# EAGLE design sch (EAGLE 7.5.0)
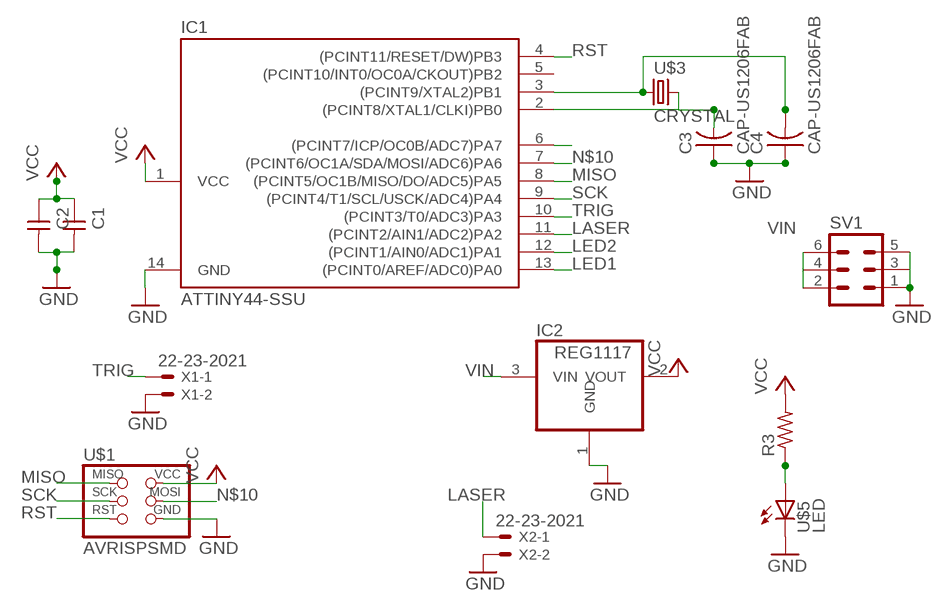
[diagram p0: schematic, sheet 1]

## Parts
C1  CAP-UNPOLARIZEDFAB  [C1206FAB]
C2  CAP-UNPOLARIZEDFAB  [C1206FAB]
C3  CAP-US1206FAB  [C1206FAB]
C4  CAP-US1206FAB  [C1206FAB]
IC1  ATTINY44-SSU  [SOIC14]
IC2  REG1117  [SOT223]
R3  RES-US1206FAB  [R1206FAB]
SV1  MA03-2  [MA03-2]
U$1  AVRISPSMD  [2X03SMD]
U$3  CRYSTAL  [2-SMD-5X3MM]
U$5  LED  [LED1206]
X1  22-23-2021  [22-23-2021]
X2  22-23-2021  [22-23-2021]

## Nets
GND: IC2.1(GND) SV1.1 SV1.3 SV1.5 X1.2 X2.2
K1: IC1.6((PCINT7/ICP/OC0B/ADC7)PA7) R3.1 U$5.1(A)
LASER: IC1.11((PCINT2/AIN1/ADC2)PA2) X2.1
LED1: IC1.13((PCINT0/AREF/ADC0)PA0)
LED2: IC1.12((PCINT1/AIN0/ADC1)PA1)
MISO: IC1.8((PCINT5/OC1B/MISO/DO/ADC5)PA5) U$1.1(MISO)
N$3: C4.2 IC1.3((PCINT9/XTAL2)PB1) U$3.P$1
N$5: C3.2 IC1.2((PCINT8/XTAL1/CLKI)PB0) U$3.P$2
N$6: C1.2 C2.2 C3.1 C4.1 IC1.14(GND) U$1.6(GND) U$5.2(C) ; supply symbol labelled GND
N$9: C1.1 C2.1 IC1.1(VCC) IC2.2(VOUT) R3.2 U$1.2(VCC) ; supply symbol labelled VCC
N$10: IC1.7((PCINT6/OC1A/SDA/MOSI/ADC6)PA6) U$1.4(MOSI)
RST: IC1.4((PCINT11/RESET/DW)PB3) U$1.5(RST)
SCK: IC1.9((PCINT4/T1/SCL/USCK/ADC4)PA4) U$1.3(SCK)
TRIG: IC1.10((PCINT3/T0/ADC3)PA3) X1.1
VIN: IC2.3(VIN) SV1.2 SV1.4 SV1.6
Unconnected: IC1.5((PCINT10/INT0/OC0A/CKOUT)PB2)

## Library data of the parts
C1 C2 = fab:CAP-UNPOLARIZED
C3 C4 = fab:CAP-US
IC1 = fab:ATTINY44
IC2 = burr-brown:REG1117: 800mA and 1A Low Dropout (LDO) Positive Regulator 1.8V, 2.5V, 2.85V, 3.3V, 5V, and Adj; MPN: REG1117; OC_FARNELL: 1097566; OC_NEWARK: 14P6981
R3 = fab:RES-US: Resistor (US Symbol)
SV1 = con-lstb:MA03-2: PIN HEADER; OC_FARNELL: unknown; OC_NEWARK: unknown
U$1 = fab:AVRISP
U$3 = fab:CRYSTAL
U$5 = fab:LED: LED
X1 X2 = con-molex:22-23-2021: .100" (2.54mm) Center Header - 2 Pin; MF: MOLEX; MPN: 22-23-2021; OC_FARNELL: 1462926; OC_NEWARK: 25C3832

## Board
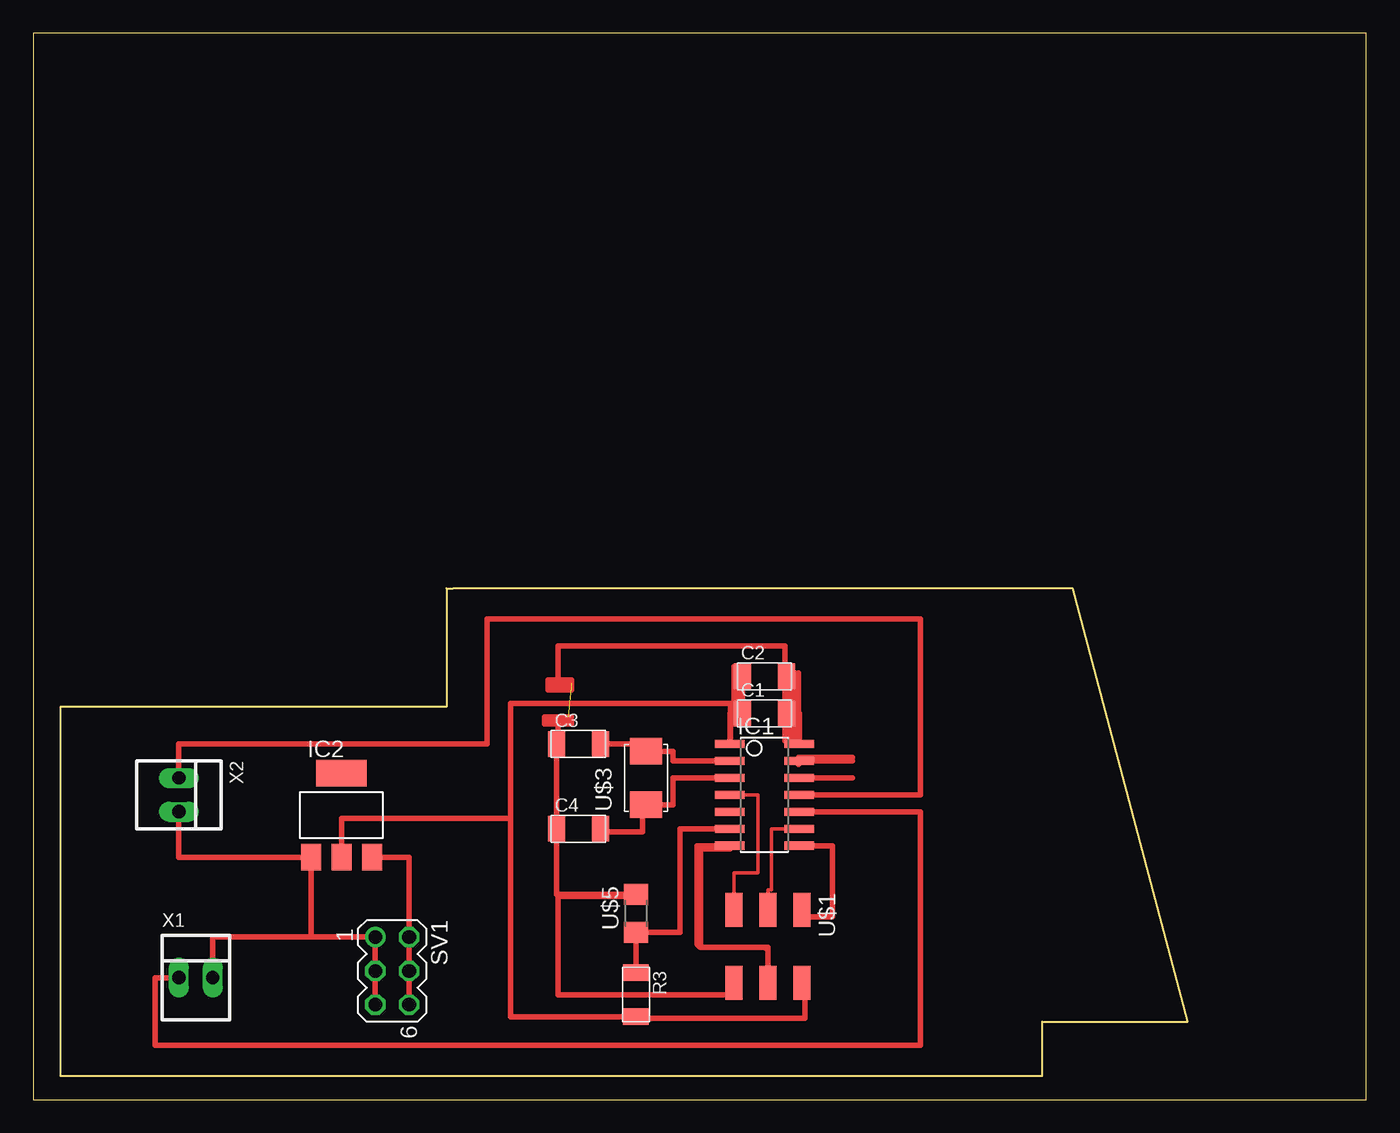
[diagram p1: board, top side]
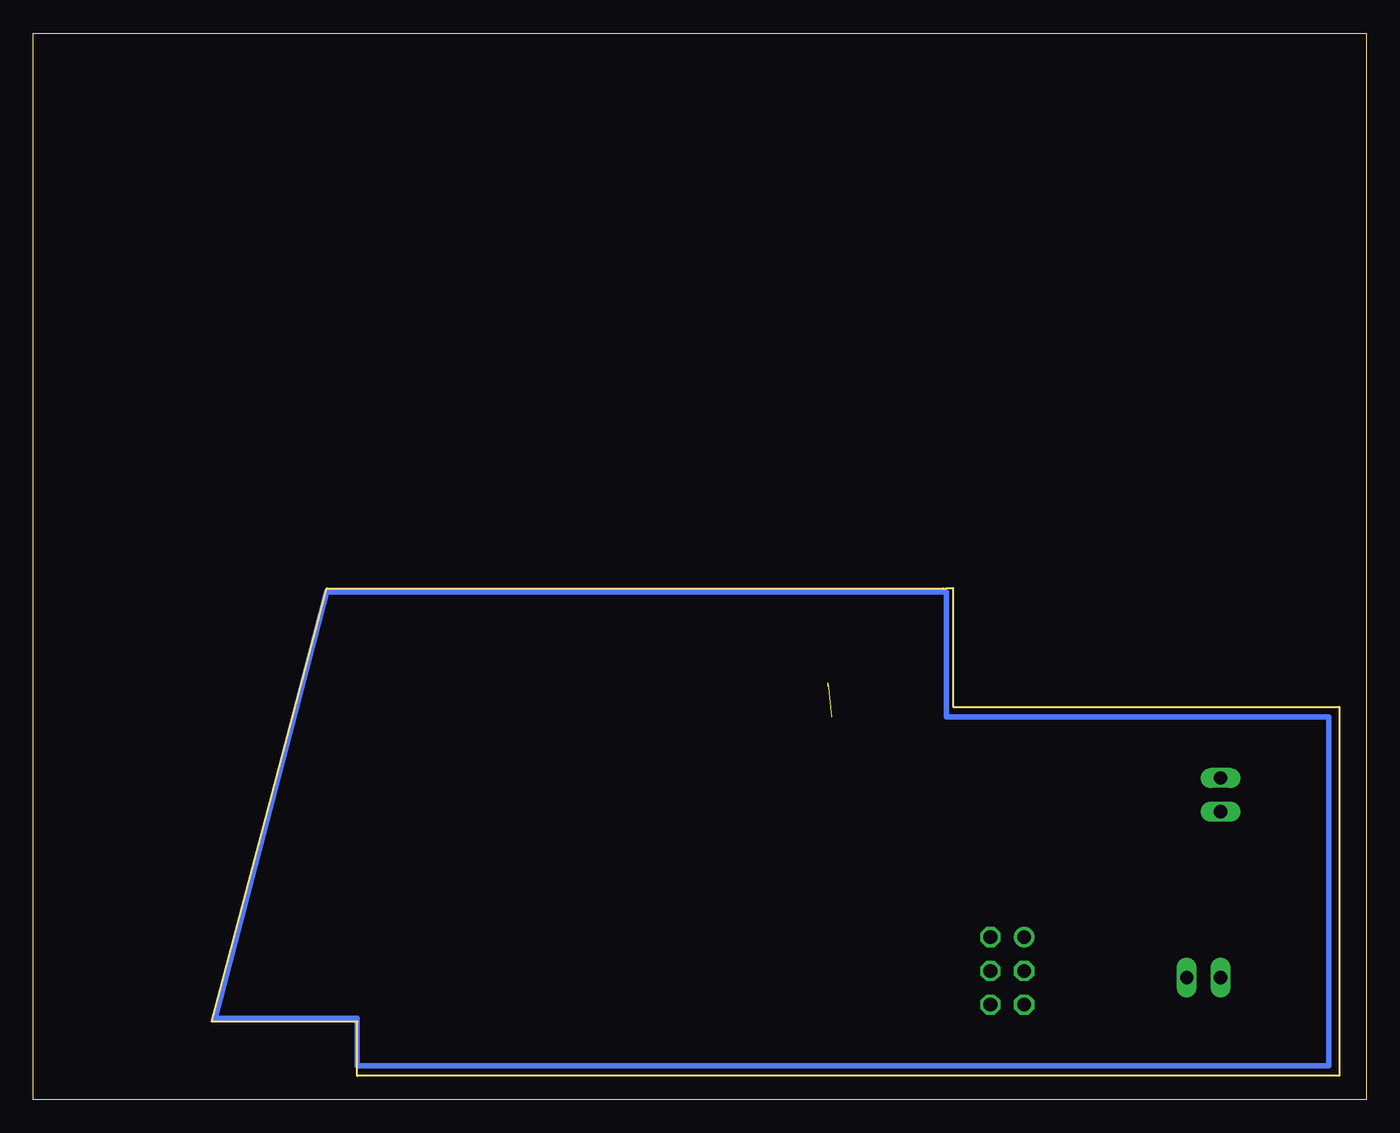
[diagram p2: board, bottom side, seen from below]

Size 100 x 80 mm. Coordinates in mm from the lower left corner, seen from the top.
Outline: 0,0 100,0 100,80 0,80 0,0
Copper layers (1*16): Top 0.035mm / dielectric 1.5mm / Bottom 0.035mm
Design rules "default": minimum track width 10mil, minimum drill 24mil, track to track 8mil, track to pad 8mil, pad to pad 8mil, via to via 8mil, smd to smd 8mil, copper to edge 40mil, drill to drill 8mil, minimum pad ring 10mil, minimum via ring 8mil, stop-mask expansion 4mil, vias tented up to drill 0mil, thermal gap 10mil
Milling: 10 lines

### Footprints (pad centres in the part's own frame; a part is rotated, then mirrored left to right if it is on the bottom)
C1206FAB = smd 1.27 x 1.905: 1 -1.651,0; 2 1.651,0
SOIC14 = smd 0.61 x 2.21: 1 -3.81,-2.603; 2 -2.54,-2.603; 3 -1.27,-2.603; 4 0,-2.603; 5 1.27,-2.603; 6 2.54,-2.603; 7 3.81,-2.603; 8 3.81,2.603; 9 2.54,2.603; 10 1.27,2.603; 11 0,2.603; 12 -1.27,2.603; 13 -2.54,2.603; 14 -3.81,2.603
SOT223 = smd 1.499 x 2.007: 1 -2.261,-3.15; 2 0.025,-3.15; 3 2.311,-3.15 | smd 3.81 x 2.007: 4 0,3.15
R1206FAB = smd 1.27 x 1.905: 1 -1.651,0; 2 1.651,0
MA03-2 = drill 1.016: 1 -2.54,-1.27 | drill 1.016 octagon: 2 -2.54,1.27; 3 0,-1.27; 4 0,1.27; 5 2.54,-1.27; 6 2.54,1.27
2X03SMD = smd 2.54 x 1.27: 1 -2.54,2.54; 2 2.92,2.54; 3 -2.54,0; 4 2.92,0; 5 -2.54,-2.54; 6 2.92,-2.54
2-SMD-5X3MM = smd 2 x 2.4: P$1 -2,0; P$2 2,0
LED1206 = smd 1.6 x 1.803: 1 -1.422,0; 2 1.422,0
22-23-2021 = drill 1 long: 1 -1.27,0; 2 1.27,0

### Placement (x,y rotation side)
C1  54.86,28.96 0 top
C2  54.86,31.75 0 top
C3  40.89,26.67 0 top
C4  40.89,20.32 0 top
IC1  54.86,22.86 270 top
IC2  23.11,21.34 0 top
R3  45.21,7.87 270 top
SV1  26.92,9.65 270 top
U$1  55.12,11.68 270 top
U$3  45.97,24.13 90 top
U$5  45.21,13.97 90 top
X1  12.19,9.14 0 top
X2  10.92,22.86 270 top

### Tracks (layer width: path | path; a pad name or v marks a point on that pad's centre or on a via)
GND
  Top 0.406: SV1.5 SV1.3 SV1.1 20.85,12.19 | 20.85,12.19 IC2.1 10.92,18.19 X2.2 | 20.85,12.19 13.46,12.19 X1.2
K1
  Top 0.406: R3.1 U$5.1 48.51,12.55 48.51,20.32 IC1.6
LASER
  Top 0.406: X2.1 10.92,26.67 34.04,26.67 34.04,36.07 66.55,36.07 66.55,22.86 IC1.11
MISO
  Top 0.406: IC1.8 59.94,19.05 59.94,13.72 57.66,13.72 U$1.1
N$3
  Top 0.406: IC1.3 48.01,24.13 48.01,22.1 45.97,22.1 U$3.P$1 45.72,22.13 45.72,20.07 42.55,20.07 C4.2
N$4
  Top 0.406: 57.66,25.4 60.45,25.4 | 61.47,25.4 60.45,25.4 | 60.45,25.4 60.45,25.65 | 60.45,25.65 61.47,25.65 | 60.45,25.65 57.4,25.65 57.4,25.15
N$5
  Top 0.406: C3.2 45.97,26.67 U$3.P$2 48.01,26.13 48.01,25.4 IC1.2
N$6  (2 unrouted)
  Top 0.406: 57.4,28.45 56.9,28.45 56.9,30.23 | 56.9,31.5 56.9,32 57.15,32 57.15,31.5 | 57.15,30.99 57.4,30.99 57.4,29.21 57.15,29.21 | C2.2 C1.2 56.64,28.96 | U$1.6 52.32,8.76 52.32,7.87 39.37,7.87 39.37,15.24 45.21,15.24 U$5.2 39.24,15.39 C4.1 C3.1 39.37,26.67 39.37,28.19 | 57.15,28.96 57.47,28.96 IC1.14 57.15,26.67 57.15,28.96 | 56.9,28.96 56.64,28.96 | 56.64,28.96 56.64,32 56.39,32 | 56.39,32 56.39,32.26 | 56.39,32.26 56.39,34.04 39.37,34.04 39.37,31.5 | 39.37,31.5 40.13,31.5 | 39.37,31.5 38.86,31.5 38.86,30.99 40.13,30.99 | 40.13,30.99 40.13,31.24 39.12,31.24 | 38.35,28.45 38.35,28.19 39.37,28.19 | 38.35,28.45 40.13,28.45 | 40.13,28.45 40.13,28.19 | 40.13,28.19 39.37,28.19 | 38.35,28.45 38.35,28.7 40.13,28.7 | 40.39,28.7 40.13,28.7 | 40.13,28.7 40.13,28.45 | 40.13,28.45 40.39,28.45 40.39,28.19 40.13,28.19 | 40.13,30.99 40.39,30.99 | 40.39,30.99 40.39,31.5 38.61,31.5 38.61,30.73 40.39,30.73 40.39,30.99 | 57.15,29.21 57.15,28.96 | 57.15,28.96 56.9,28.96 | 56.9,28.96 56.9,26.92 | 57.15,30.99 57.15,29.21 | 57.15,30.99 57.15,31.5 | 57.15,31.5 56.39,32.26 | 56.39,32 56.39,26.92 56.64,26.92 56.64,29.97 56.9,30.23 | 56.9,30.23 56.9,31.5 | 56.9,31.5 57.4,32 57.4,27.94
N$7
  Top 0.406: 61.47,24.13 57.66,24.13
N$8
  Bottom 0.406: 75.69,6.1 86.36,6.1 77.98,38.1 31.5,38.1 31.5,28.7 2.79,28.7 2.79,2.54 75.69,2.54 75.69,6.1
N$9
  Top 0.406: 53.09,28.19 52.58,28.19 52.58,28.96 | 53.59,31.75 C2.1 C1.1 52.83,28.96 | U$1.2 57.91,8.76 57.91,6.1 45.21,6.1 R3.2 35.81,6.22 35.81,21.08 | 52.58,28.96 52.26,28.96 IC1.1 52.32,26.67 52.32,29.72 35.81,29.72 35.81,21.08 | 35.81,21.08 23.14,21.08 IC2.2 | 52.83,32.51 52.83,28.96 | 52.83,28.96 52.58,28.96 | 52.58,28.96 52.58,32.51 53.09,32.51 53.09,30.73
N$10
  Top 0.406: 52.58,19.05 49.78,19.05 49.78,11.68 50.04,11.43 | 55.12,11.18 55.12,11.43 54.86,11.43 | 50.04,11.43 50.04,18.8 52.26,18.8 IC1.7 | 50.04,11.43 54.86,11.43 | 54.86,11.43 55.12,11.18 | 55.12,11.18 U$1.4
RST
  Top 0.254: IC1.4 54.36,22.86 54.36,17.02 52.58,17.02 U$1.5
SCK
  Top 0.254: IC1.9 55.37,20.32 55.37,15.75 55.12,15.75 U$1.3
TRIG
  Top 0.406: X1.1 9.14,9.14 9.14,4.06 66.55,4.06 66.55,21.59 IC1.10
VIN
  Top 0.406: IC2.3 28.19,18.19 SV1.2 SV1.4 SV1.6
